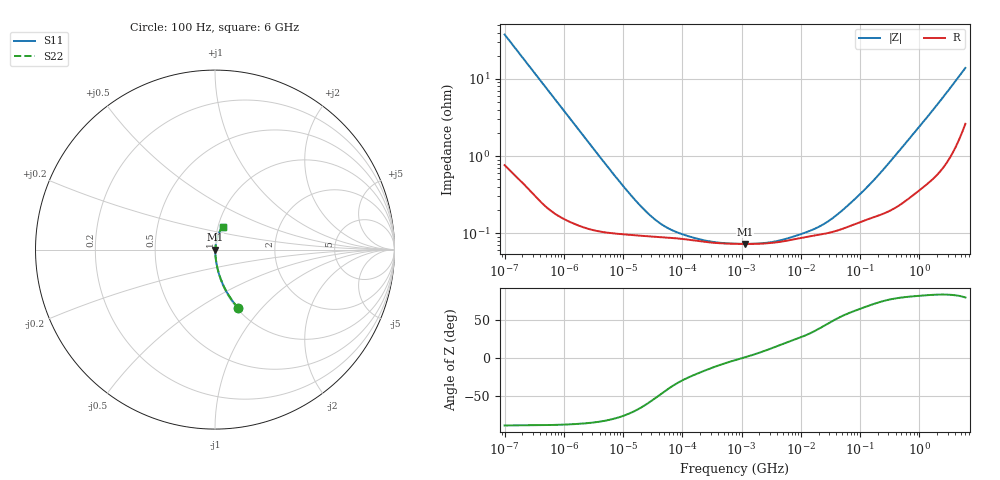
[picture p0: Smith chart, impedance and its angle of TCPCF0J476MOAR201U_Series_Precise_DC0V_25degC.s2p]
! TCPCF0J476MOAR201U Polymer Tantalum Capacitor Sparameter Model
! Model Generated by Samsung Electro-Mechanics
! Samsung Sparameter Version 5.0
! Date : Oct-10-2024
! Products : Polymer Tantalum Capacitor
! Characteristics :
!  Nominal Capacitance = 47uF
!  Capacitance Tolerance = +/-20%
!  ESR = 200 mohm max at 100kHz
!  Rated Voltage = 6.3Vdc
!  Size = 0805(unit:inch), 2012(unit:mm)
!  Length = 2.00+/-0.20mm
!  Width = 1.25+/-0.20mm
!  Thickness = 0.70+/-0.10mm
!  Lineup = Conductive Polymer Type
!  Feature = PCF
!  Measurement Temperature : 25degC.
!  DC bias Value = 0V
!  Frequency : 100Hz ~ 6GHz
! External Node Assignments :
!  1  o---||---o  2
# MHz S RI R 50.0
! Freq.  Real(S11)  Im(S11)  Real(S12)  Im(S12)  Real(S21)  Im(S21)  Real(S22)  Im(S22)
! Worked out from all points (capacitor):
!   300 points, 100 Hz to 6 GHz, reference 50 ohm
!   read as one part in series: C = 42.1 uF near 106.2 Hz
!   lowest |Z| = 72.6 mohm at 1.143 MHz (marker M1)
!   series resonance near 1.067 MHz, so ESL is about 530 pH
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0.0001  0.1295 -0.3258  0.8705 0.3258  0.8705 0.3258  0.1295 -0.3258
0.0001714451  0.0511 -0.2091  0.9489 0.2091  0.9489 0.2091  0.0511 -0.2091
0.0003517965  0.0145 -0.1071  0.9855 0.1071  0.9855 0.1071  0.0145 -0.1071
0.0007664292  0.00424 -0.0501  0.9958 0.0501  0.9958 0.0501  0.00424 -0.0501
0.001998454  0.00159 -0.0195  0.9984 0.0195  0.9984 0.0195  0.00159 -0.0195
0.01358747  0.000956 -0.00294  0.999 0.00294  0.999 0.00294  0.000956 -0.00294
0.02473303  0.000917 -0.00165  0.9991 0.00165  0.9991 0.00165  0.000917 -0.00165
0.03993819  0.000894 -0.00105  0.9991 0.00105  0.9991 0.00105  0.000894 -0.00105
0.0726988  0.000863 -0.00062  0.9991 0.00062  0.9991 0.00062  0.000863 -0.00062
0.1583827  0.000803 -0.000332  0.9992 0.000332  0.9992 0.000332  0.000803 -0.000332
0.3450549  0.000749 -0.00016  0.9993 0.00016  0.9993 0.00016  0.000749 -0.00016
0.7981464  0.000727 -3.63e-05  0.9993 3.63e-05  0.9993 3.63e-05  0.000727 -3.63e-05
1.143315  0.000725 8.77e-06  0.9993 -8.77e-06  0.9993 -8.77e-06  0.000725 8.77e-06
2.209625  0.000732 0.000101  0.9993 -0.000101  0.9993 -0.000101  0.000732 0.000101
4.022142  0.000763 0.000211  0.9992 -0.000211  0.9992 -0.000211  0.000763 0.000211
15.95059  0.000923 0.000619  0.9991 -0.000619  0.9991 -0.000619  0.000923 0.000619
29.03458  0.00101 0.00101  0.999 -0.00101  0.999 -0.00101  0.00101 0.00101
56.11362  0.00117 0.00177  0.9988 -0.00177  0.9988 -0.00177  0.00117 0.00177
137.8087  0.00153 0.0038  0.9985 -0.0038  0.9985 -0.0038  0.00153 0.0038
318.7652  0.00201 0.00814  0.998 -0.00814  0.998 -0.00814  0.00201 0.00814
1922.593  0.00742 0.0436  0.9926 -0.0436  0.9926 -0.0436  0.00742 0.0436
6000  0.0425 0.1274  0.9575 -0.1274  0.9575 -0.1274  0.0425 0.1274
